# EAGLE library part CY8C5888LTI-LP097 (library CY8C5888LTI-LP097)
MCU 32-Bit CY8C58LPxxx ARM Cortex M3 RISC 256KB Flash 1.8V/3.3V/5V 68-Pin QFN EP Tray Check availability
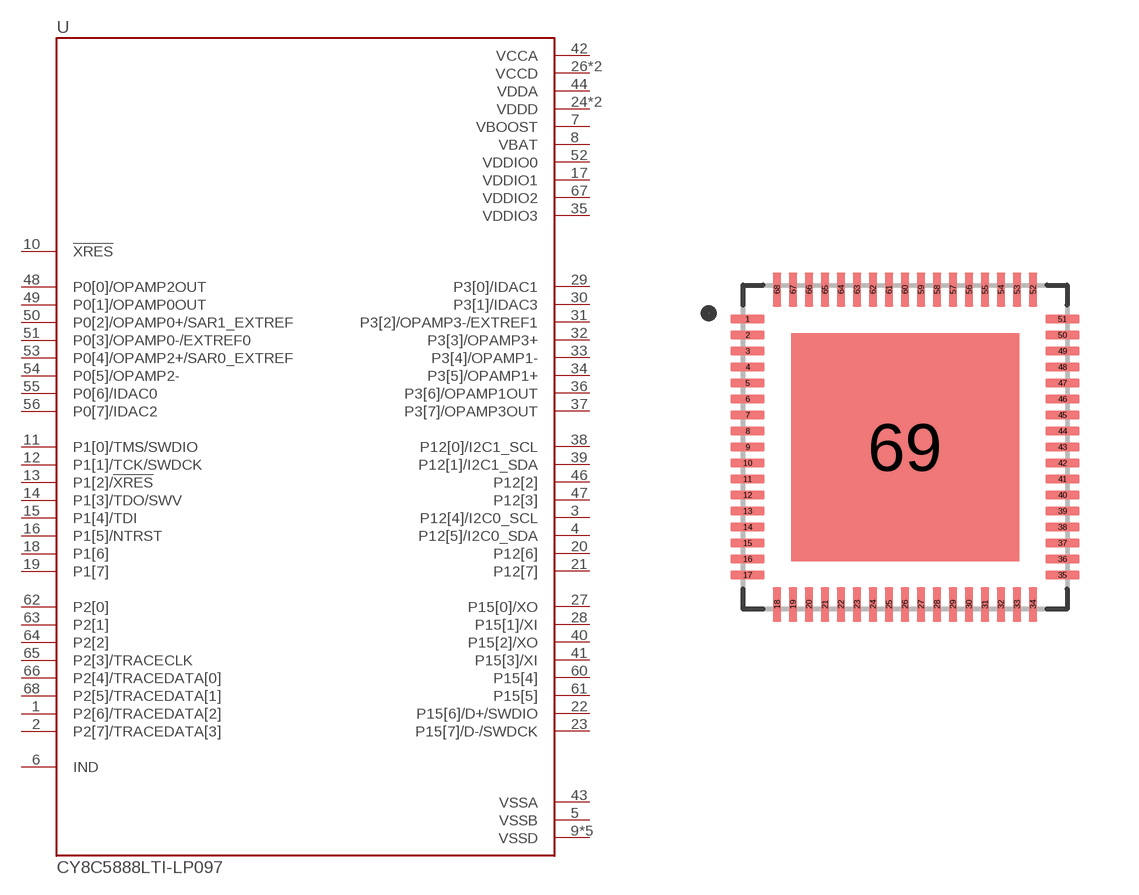
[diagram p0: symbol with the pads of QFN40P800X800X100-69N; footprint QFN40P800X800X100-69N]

Designator prefix U

## CY8C5888LTI-LP097 (Availability: In Stock; Check_prices: https://www.snapeda.com/parts/CY8C5888LTI-LP097/Cypress+semiconductor/view-part/?ref=eda; Description: ARM® Cortex®-M3 PSOC® 5 CY8C58LP Microcontroller IC 32-Bit Single-Core 80MHz 256KB (256K x 8) FLASH 68-QFN (8x8); MF: Cypress Semiconductor; MP: CY8C5888LTI-LP097; Package: VFQFN-68 Cypress Semiconductor; Price: None; SnapEDA_Link: https://www.snapeda.com/parts/CY8C5888LTI-LP097/Cypress+semiconductor/view-part/?ref=snap)  [QFN40P800X800X100-69N]
1  P2[6]/TRACEDATA[2]
2  P2[7]/TRACEDATA[3]
3  P12[4]/I2C0_SCL
4  P12[5]/I2C0_SDA
5  VSSB  pwr
6  IND  pas
7  VBOOST  pwr
8  VBAT  pwr
9  VSSD  pwr
10  !XRES  in
11  P1[0]/TMS/SWDIO
12  P1[1]/TCK/SWDCK
13  P1[2]/!XRES
14  P1[3]/TDO/SWV
15  P1[4]/TDI
16  P1[5]/NTRST
17  VDDIO1  pwr
18  P1[6]
19  P1[7]
20  P12[6]
21  P12[7]
22  P15[6]/D+/SWDIO
23  P15[7]/D-/SWDCK
24  VDDD  pwr
25  VSSD  pwr
26  VCCD  pwr
27  P15[0]/XO
28  P15[1]/XI
29  P3[0]/IDAC1
30  P3[1]/IDAC3
31  P3[2]/OPAMP3-/EXTREF1
32  P3[3]/OPAMP3+
33  P3[4]/OPAMP1-
34  P3[5]/OPAMP1+
35  VDDIO3  pwr
36  P3[6]/OPAMP1OUT
37  P3[7]/OPAMP3OUT
38  P12[0]/I2C1_SCL
39  P12[1]/I2C1_SDA
40  P15[2]/XO
41  P15[3]/XI
42  VCCA  pwr
43  VSSA  pwr
44  VDDA  pwr
45  VSSD  pwr
46  P12[2]
47  P12[3]
48  P0[0]/OPAMP2OUT
49  P0[1]/OPAMP0OUT
50  P0[2]/OPAMP0+/SAR1_EXTREF
51  P0[3]/OPAMP0-/EXTREF0
52  VDDIO0  pwr
53  P0[4]/OPAMP2+/SAR0_EXTREF
54  P0[5]/OPAMP2-
55  P0[6]/IDAC0
56  P0[7]/IDAC2
57  VCCD  pwr
58  VSSD  pwr
59  VDDD  pwr
60  P15[4]
61  P15[5]
62  P2[0]
63  P2[1]
64  P2[2]
65  P2[3]/TRACECLK
66  P2[4]/TRACEDATA[0]
67  VDDIO2  pwr
68  P2[5]/TRACEDATA[1]
69  VSSD  pwr

## Footprint QFN40P800X800X100-69N (pad centres in mm)
smd 0.86 x 0.22: 1 -3.935,3.2; 2 -3.935,2.8; 3 -3.935,2.4; 4 -3.935,2; 5 -3.935,1.6; 6 -3.935,1.2; 7 -3.935,0.8; 8 -3.935,0.4; 9 -3.935,0; 10 -3.935,-0.4; 11 -3.935,-0.8; 12 -3.935,-1.2; 13 -3.935,-1.6; 14 -3.935,-2; 15 -3.935,-2.4; 16 -3.935,-2.8; 17 -3.935,-3.2; 35 3.935,-3.2; 36 3.935,-2.8; 37 3.935,-2.4; 38 3.935,-2; 39 3.935,-1.6; 40 3.935,-1.2; 41 3.935,-0.8; 42 3.935,-0.4; 43 3.935,0; 44 3.935,0.4; 45 3.935,0.8; 46 3.935,1.2; 47 3.935,1.6; 48 3.935,2; 49 3.935,2.4; 50 3.935,2.8; 51 3.935,3.2
smd 0.22 x 0.86: 18 -3.2,-3.935; 19 -2.8,-3.935; 20 -2.4,-3.935; 21 -2,-3.935; 22 -1.6,-3.935; 23 -1.2,-3.935; 24 -0.8,-3.935; 25 -0.4,-3.935; 26 0,-3.935; 27 0.4,-3.935; 28 0.8,-3.935; 29 1.2,-3.935; 30 1.6,-3.935; 31 2,-3.935; 32 2.4,-3.935; 33 2.8,-3.935; 34 3.2,-3.935; 52 3.2,3.935; 53 2.8,3.935; 54 2.4,3.935; 55 2,3.935; 56 1.6,3.935; 57 1.2,3.935; 58 0.8,3.935; 59 0.4,3.935; 60 0,3.935; 61 -0.4,3.935; 62 -0.8,3.935; 63 -1.2,3.935; 64 -1.6,3.935; 65 -2,3.935; 66 -2.4,3.935; 67 -2.8,3.935; 68 -3.2,3.935
smd 5.7 x 5.7: 69 0,0

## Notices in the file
This work is licensed under a Creative Commons Attribution-ShareAlike 4.0 International License (CC BY-SA) with Design Exception 1.0
